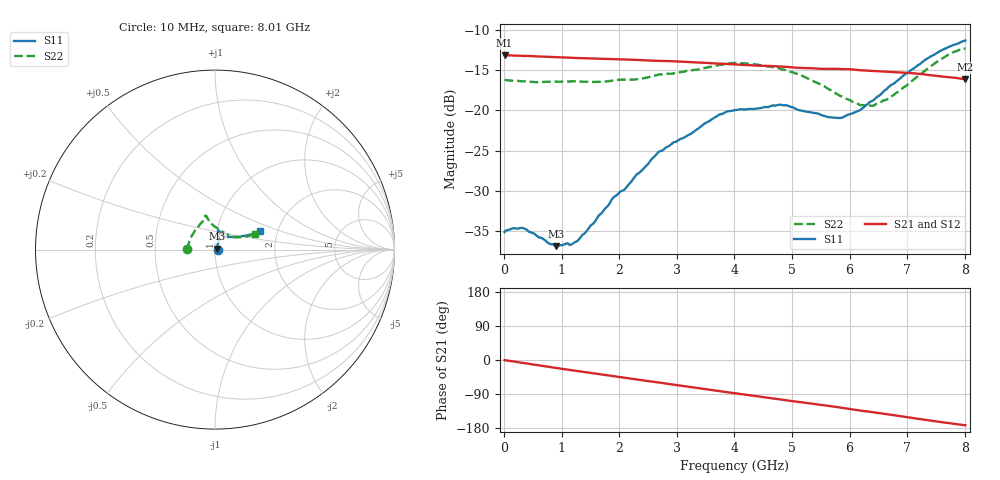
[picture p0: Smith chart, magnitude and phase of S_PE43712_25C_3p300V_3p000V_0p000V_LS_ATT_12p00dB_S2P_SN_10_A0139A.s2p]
! DEVICE ID: PE43712
! File Path: z:\PE43713\PE43713_CHAR_NOM_04292014\AMB\3p300\LS_ATT_12p00dB\PE43713_AMB_3p300V_3p000V_0p000V_LS_ATT_12p00dB_S2P_SN_10_A0139A.s2p
! Serial: 10
! Lot: A0139A
! Temp: 25C
! VDD: 3.300
! VSS: 0.000
! Control_Hi: 3.000
! Control_Lo: 0.000
! Attenuation Step: 12.00dB
! Port 1: RF1
! Port 2: RF2
! ThroughPath:1-2
! IDD: 0.0001470103
! ISS: -2.068e-007
#  Hz  S  RI  R  50
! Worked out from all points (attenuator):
!   801 points, 10 MHz to 8.01 GHz, reference 50 ohm
!   highest |S21| = -13.19 dB at 10 MHz (marker M1); lowest = -16.1 dB at 8.01 GHz (marker M2)
!   lowest |S11| = -36.8 dB at 910 MHz (marker M3), VSWR 1.03, Z = 51.4 + j0.517 ohm
!   |S11| at or under -10 dB: start of sweep to end of sweep
!   |S22| runs from -19.5 to -12.3 dB; largest |S21 - S12| = 0.0008
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1e7  0.0176 0.000276  0.219 -0.00118  0.2192 -0.00109  -0.1542 0.00105
1.6e8  0.0186 0.000618  0.2178 -0.0151  0.218 -0.0151  -0.152 0.0105
3.4e8  0.0186 0.000298  0.2148 -0.0312  0.2148 -0.0307  -0.1499 0.0193
9.1e8  0.0135 0.00503  0.1987 -0.0772  0.1989 -0.0773  -0.1421 0.0495
1.18e9  0.0115 0.00931  0.188 -0.0961  0.188 -0.0962  -0.1367 0.0641
1.35e9  0.0117 0.012  0.1807 -0.1074  0.1808 -0.1075  -0.1322 0.0719
1.9e9  0.0137 0.0254  0.1527 -0.1402  0.1527 -0.1402  -0.1142 0.102
2.11e9  0.0148 0.0293  0.1404 -0.151  0.1405 -0.151  -0.108 0.111
2.68e9  0.023 0.0501  0.1033 -0.1739  0.1033 -0.174  -0.0813 0.1451
3.72e9  0.0237 0.09  0.0284 -0.1926  0.0283 -0.1926  -0.0558 0.1817
4.01e9  0.0221 0.0979  0.00758 -0.1924  0.00753 -0.1923  -0.0551 0.1885
4.79e9  0.0198 0.1066  -0.045 -0.1811  -0.045 -0.1813  -0.0429 0.1761
5.35e9  0.0302 0.0918  -0.078 -0.1644  -0.078 -0.1643  -0.0282 0.1507
5.64e9  0.0406 0.0811  -0.0933 -0.1546  -0.0933 -0.1547  -0.00936 0.1347
5.88e9  0.0514 0.0742  -0.1071 -0.1448  -0.1068 -0.1448  0.00967 0.1209
6.17e9  0.0705 0.0706  -0.1209 -0.1296  -0.1207 -0.1298  0.0379 0.1013
6.3e9  0.0829 0.0697  -0.1258 -0.1231  -0.1256 -0.123  0.0523 0.0928
6.42e9  0.0927 0.0696  -0.1303 -0.1169  -0.1301 -0.1169  0.0648 0.0854
6.68e9  0.1201 0.0707  -0.1395 -0.1022  -0.1392 -0.1022  0.0938 0.0736
7.36e9  0.1929 0.0837  -0.1546 -0.0592  -0.1545 -0.0592  0.1663 0.0725
7.72e9  0.2283 0.0937  -0.1558 -0.0373  -0.1557 -0.0374  0.2056 0.082
8.01e9  0.2494 0.1051  -0.1544 -0.0213  -0.1543 -0.0215  0.2249 0.0876
